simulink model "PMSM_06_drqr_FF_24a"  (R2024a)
settings: Solver=ode45  StartTime=0.0  StopTime=0.1  MaxStep=1e-4  RelTol=1e-4  AbsTol=1e-4  EnableMultiTasking=on
undefined symbols (not defined in the file): by, established, Flux, linkage, magnets, V
libraries: spsControlledVoltageSourceLib x3, spsCurrentMeasurementLib x3, slpidlib x2, spsPermanentMagnetSynchronousMachineLib x1, spspowerguiLib x1

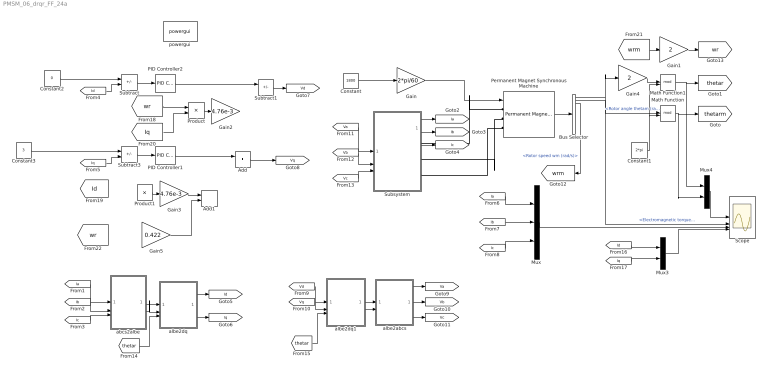
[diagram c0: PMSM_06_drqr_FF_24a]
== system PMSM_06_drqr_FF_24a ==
  Add : Sum
  Add1 : Sum
  Bus Selector : BusSelector  OutputSignals=Rotor angle thetam (rad),Electromagnetic torque Te (N*m),Rotor speed wm (rad/s)
  Constant : Constant  Value=1800
  Constant1 : Constant  Value=2*pi
  Constant2 : Constant  Value=0
  Constant3 : Constant  Value=3
  Gain : Gain  Gain=2*pi/60
  Gain1 : Gain  Gain=2
  Gain2 : Gain  Gain=4.76e-3
  Gain3 : Gain  Gain=4.76e-3
  Gain4 : Gain  Gain=2
  Gain5 : Gain  Gain=0.422
  Math Function : Math  Operator=mod  SignedPower=on
  Math Function1 : Math  Operator=mod  SignedPower=on
  Mux : Mux  Inputs=3
  Mux3 : Mux  Inputs=2
  Mux4 : Mux  Inputs=2
  PID Controller1 : slpidlib/PID Controller  Controller=PI  Form=Parallel  TimeDomain=Continuous-time  UseExternalTs=off  SampleTime=1  IntegratorMethod=Forward Euler  FilterMethod=Forward Euler  ControllerParametersSource=internal  P=14.95  I=1328.9  UseKiTs=off  D=0  UseExternalDerivativeSource=off  N=100  UseFilter=on  TunerSelectOption=Transfer Function Based (PID Tuner App)  InitialConditionSource=internal  InitialConditionForIntegrator=0  InitialConditionForFilter=0  DifferentiatorICPrevScaledInput=0  ExternalReset=none  TrackingMode=off  Kt=1  LimitOutput=off  SatLimitsSource=internal  UpperSaturationLimit=inf  LowerSaturationLimit=-inf  LinearizeAsGain=on  AntiWindupMode=none  Kb=1  LimitIntegrator=off  UpperIntegratorSaturationLimit=inf  LowerIntegratorSaturationLimit=-inf  POutMin=[]  POutMax=[]  IOutMin=[]  IOutMax=[]  DOutMin=[]  DOutMax=[]  NOutMin=[]  NOutMax=[]  SumOutMin=[]  SumOutMax=[]  SaturationOutMin=[]  SaturationOutMax=[]  PParamMin=[]  PParamMax=[]  IParamMin=[]  IParamMax=[]  DParamMin=[]  DParamMax=[]  NParamMin=[]  NParamMax=[]  KbParamMin=[]  KbParamMax=[]  KtParamMin=[]  KtParamMax=[]  KbOutMin=[]  KbOutMax=[]  KtOutMin=[]  KtOutMax=[]  IntegratorOutMin=[]  IntegratorOutMax=[]  FilterOutMin=[]  FilterOutMax=[]  SumI1OutMin=[]  SumI1OutMax=[]  SumI2OutMin=[]  SumI2OutMax=[]  SumI3OutMin=[]  SumI3OutMax=[]  SumI4OutMin=[]  SumI4OutMax=[]  SumDOutMin=[]  SumDOutMax=[]  DifferentiatorOutMin=[]  DifferentiatorOutMax=[]  FilterDiffOutCoefMin=[]  FilterDiffOutCoefMax=[]  ReciprocalOutMin=[]  ReciprocalOutMax=[]  SumDenOutMin=[]  SumDenOutMax=[]  SumNumOutMin=[]  SumNumOutMax=[]  DivideOutMin=[]  DivideOutMax=[]  UdiffTsProdOutMin=[]  UdiffTsProdOutMax=[]  NTsProdOutMin=[]  NTsProdOutMax=[]  UintegralTsProdOutMin=[]  UintegralTsProdOutMax=[]  UngainTsProdOutMin=[]  UngainTsProdOutMax=[]  ClampingZeroOutDataTypeStr=Inherit: Inherit via back propagation  ClampingZeroOutMin=[]  ClampingZeroOutMax=[]  FilterDenConstantOutDataTypeStr=Inherit: Inherit via back propagation  FilterDenConstantOutMin=[]  FilterDenConstantOutMax=[]  PCopyOutDataTypeStr=Inherit: Inherit via back propagation  PCopyOutMin=[]  PCopyOutMax=[]  NCopyOutDataTypeStr=Inherit: Inherit via back propagation  NCopyOutMin=[]  NCopyOutMax=[]  IntegratorContinuousStateAttributes=''  IntegratorStateMustResolveToSignalObject=off  IntegratorRTWStateStorageClass=Auto  FilterContinuousStateAttributes=''  FilterStateMustResolveToSignalObject=off  FilterRTWStateStorageClass=Auto  ParallelPVariant=InternalParameters  IdealPVariant=Disabled  IVariant=InternalParameters  DVariant=Disabled  IntegratorVariant=Continuous  SatVariant=Disabled  AWVariant=Passthrough  PCopyVariant=Disabled  TRVariant=Disabled  FdbkBlocksVariant=Forward  IdealPFdbkVariant=Disabled  SatFdbkVariant=Disabled  DerivativeFilterVariant=Disabled  NVariant=Disabled  NCopyVariant=Disabled_SignalSpec  FilterICVariant=Disabled  IntegratorICVariant=InternalICs  ExternalResetVariant=Disabled  TRSumVariant=Passthrough  SumFdbkVariant=Disabled  SumVariant=Sum_PI  TsampFilterVariant=InternalTs  TsampNgainVariant=Passthrough  TsampIntegralVariant=Disabled_SignalSpec  ExternalSaturationOutDataTypeStr=Inherit: Same as second input  DerivativeSourceVariant=Disabled
  PID Controller2 : slpidlib/PID Controller  Controller=PI  Form=Parallel  TimeDomain=Continuous-time  UseExternalTs=off  SampleTime=1  IntegratorMethod=Forward Euler  FilterMethod=Forward Euler  ControllerParametersSource=internal  P=14.95  I=1328.9  UseKiTs=off  D=0  UseExternalDerivativeSource=off  N=100  UseFilter=on  TunerSelectOption=Transfer Function Based (PID Tuner App)  InitialConditionSource=internal  InitialConditionForIntegrator=0  InitialConditionForFilter=0  DifferentiatorICPrevScaledInput=0  ExternalReset=none  TrackingMode=off  Kt=1  LimitOutput=off  SatLimitsSource=internal  UpperSaturationLimit=inf  LowerSaturationLimit=-inf  LinearizeAsGain=on  AntiWindupMode=none  Kb=1  LimitIntegrator=off  UpperIntegratorSaturationLimit=inf  LowerIntegratorSaturationLimit=-inf  POutMin=[]  POutMax=[]  IOutMin=[]  IOutMax=[]  DOutMin=[]  DOutMax=[]  NOutMin=[]  NOutMax=[]  SumOutMin=[]  SumOutMax=[]  SaturationOutMin=[]  SaturationOutMax=[]  PParamMin=[]  PParamMax=[]  IParamMin=[]  IParamMax=[]  DParamMin=[]  DParamMax=[]  NParamMin=[]  NParamMax=[]  KbParamMin=[]  KbParamMax=[]  KtParamMin=[]  KtParamMax=[]  KbOutMin=[]  KbOutMax=[]  KtOutMin=[]  KtOutMax=[]  IntegratorOutMin=[]  IntegratorOutMax=[]  FilterOutMin=[]  FilterOutMax=[]  SumI1OutMin=[]  SumI1OutMax=[]  SumI2OutMin=[]  SumI2OutMax=[]  SumI3OutMin=[]  SumI3OutMax=[]  SumI4OutMin=[]  SumI4OutMax=[]  SumDOutMin=[]  SumDOutMax=[]  DifferentiatorOutMin=[]  DifferentiatorOutMax=[]  FilterDiffOutCoefMin=[]  FilterDiffOutCoefMax=[]  ReciprocalOutMin=[]  ReciprocalOutMax=[]  SumDenOutMin=[]  SumDenOutMax=[]  SumNumOutMin=[]  SumNumOutMax=[]  DivideOutMin=[]  DivideOutMax=[]  UdiffTsProdOutMin=[]  UdiffTsProdOutMax=[]  NTsProdOutMin=[]  NTsProdOutMax=[]  UintegralTsProdOutMin=[]  UintegralTsProdOutMax=[]  UngainTsProdOutMin=[]  UngainTsProdOutMax=[]  ClampingZeroOutDataTypeStr=Inherit: Inherit via back propagation  ClampingZeroOutMin=[]  ClampingZeroOutMax=[]  FilterDenConstantOutDataTypeStr=Inherit: Inherit via back propagation  FilterDenConstantOutMin=[]  FilterDenConstantOutMax=[]  PCopyOutDataTypeStr=Inherit: Inherit via back propagation  PCopyOutMin=[]  PCopyOutMax=[]  NCopyOutDataTypeStr=Inherit: Inherit via back propagation  NCopyOutMin=[]  NCopyOutMax=[]  IntegratorContinuousStateAttributes=''  IntegratorStateMustResolveToSignalObject=off  IntegratorRTWStateStorageClass=Auto  FilterContinuousStateAttributes=''  FilterStateMustResolveToSignalObject=off  FilterRTWStateStorageClass=Auto  ParallelPVariant=InternalParameters  IdealPVariant=Disabled  IVariant=InternalParameters  DVariant=Disabled  IntegratorVariant=Continuous  SatVariant=Disabled  AWVariant=Passthrough  PCopyVariant=Disabled  TRVariant=Disabled  FdbkBlocksVariant=Forward  IdealPFdbkVariant=Disabled  SatFdbkVariant=Disabled  DerivativeFilterVariant=Disabled  NVariant=Disabled  NCopyVariant=Disabled_SignalSpec  FilterICVariant=Disabled  IntegratorICVariant=InternalICs  ExternalResetVariant=Disabled  TRSumVariant=Passthrough  SumFdbkVariant=Disabled  SumVariant=Sum_PI  TsampFilterVariant=InternalTs  TsampNgainVariant=Passthrough  TsampIntegralVariant=Disabled_SignalSpec  ExternalSaturationOutDataTypeStr=Inherit: Same as second input  DerivativeSourceVariant=Disabled
  Permanent Magnet Synchronous Machine : spsPermanentMagnetSynchronousMachineLib/Permanent Magnet Synchronous Machine  NbPhases=3  FluxDistribution=Sinusoidal  RotorType=Round  MechanicalLoad=Speed w  PresetModel=No  ShowDetailedParameters=on  MeasurementBus=off  Resistance=0.423  Inductance=8.5e-3  dqInductances=[8.5e-3,8.5e-3]  La=0.00476  MachineConstant=Flux linkage established by magnets (V.s)  Flux=0.422  VoltageCst=153.0847  TorqueCst=1.266  Flat=120  Mechanical=[0.03 0.04 4 0]  PolePairs=2  InitialConditions=[0,0, 0,0]  InitialConditions5ph=[0 0 0 0 0 0]  RefAngle=Aligned with phase A axis (original Park)  IterativeDiscreteModel=Trapezoidal non iterative  TsBlock=-1  TsPowergui=0
  Product : Product
  Product1 : Product
  Scope : Scope  NumInputPorts=4
  Subsystem : Subsystem
  Subtract : Sum  Inputs=+-
  Subtract1 : Sum  Inputs=+-
  Subtract3 : Sum  Inputs=+-
  abcs2albe : Subsystem
  albe2abcs : Subsystem
  albe2dq : Subsystem
  albe2dq1 : Subsystem
  powergui : spspowerguiLib/powergui  Priority=1  SimulationMode=Continuous  SampleTime=50e-6  frequency=60  Iterations=50  frequencyindice=0  Pbase=100e6  ErrMax=1e-4  UnitsV=kV  UnitsW=MW  buscounter=0  FunctionMessages=off  echomessages=off  EnableUseOfTLC=off  CurrentSourceSwitches=off  DisableSnubberDevices=on  DisableRonSwitches=on  DisableVfSwitches=on  DisplayEquations=off  AutomaticDiscreteSolvers=off  SolverType=Tustin  Interpol=off  ExternalGateDelay=off  methode=off  Ts=0  x0status=blocks  SPID=on  SwTol=0  HookPort=off  NonlinearTolerance=1e-4  nMaxIteration=100  ContinueOnMaxIteration=off  RestoreLinks=warning  ResistiveCurrentMeasurement=off  Frange=[0:2:500]  Ylog=off  Xlog=on  ShowGrid=off  save=off  variable=ZData  structure=0  ZoomFFT=off  StartTime=0.0  cycles=1  DisplayStyle=1  fundamental=60  FreqAxis=off  MaxFrequency=1000  frequencyindicesteady=1  RmsSteady=1  display=off
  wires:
  Gain/1 -> Permanent Magnet Synchronous Machine/1
  Constant/1 -> Gain/1
  Subtract/1 -> PID Controller2/1
  Permanent Magnet Synchronous Machine/1 -> Bus Selector/1
  Mux/1 -> Scope/3
  Bus Selector/2 -> Scope/2  "<Electromagnetic torque Te (N*m)>"
  Bus Selector/1 -> Gain4/1, Math Function/1  "<Rotor angle thetam (rad)>"
  Constant1/1 -> Math Function1/2, Math Function/2
  Math Function/1 -> Mux4/2, [thetarm]
  Gain4/1 -> Math Function1/1
  Math Function1/1 -> Mux4/1, [thetar]
  Subtract3/1 -> PID Controller1/1
  Subsystem/1(Out1) -> [Ia]
  Subsystem/2(Out2) -> [Ib]
  Subsystem/3(Out3) -> [Ic]
  [Id] -> Subtract/2
  [Iq] -> Subtract3/2
  [Ia] -> Mux/1
  [Ib] -> Mux/2
  [Ic] -> Mux/3
  Mux3/1 -> Scope/4
  [Id] -> Mux3/1
  [Iq] -> Mux3/2
  Mux4/1 -> Scope/1
  albe2dq1/1(alpha) -> albe2abcs/1(alpha)
  albe2dq1/2(beta) -> albe2abcs/2(beta)
  albe2abcs/1(as) -> [Va]
  albe2abcs/2(bs) -> [Vb]
  albe2abcs/3(cs) -> [Vc]
  [Ia] -> abcs2albe/1(as)
  [Ib] -> abcs2albe/2(bs)
  [Ic] -> abcs2albe/3(cs)
  [Vc] -> Subsystem/3(In3)
  [Vb] -> Subsystem/2(In2)
  [Va] -> Subsystem/1(In1)
  Bus Selector/3 -> [wrm]  "<Rotor speed wm (rad/s)>"
  abcs2albe/1(alpha) -> albe2dq/1(alpha)
  abcs2albe/2(beta) -> albe2dq/2(beta)
  albe2dq/1(d) -> [Id]
  albe2dq/2(q) -> [Iq]
  [thetar] -> albe2dq/3(thetar)
  [Vq] -> albe2dq1/2(q)
  [Vd] -> albe2dq1/1(d)
  [thetar] -> albe2dq1/3(thetar)
  Constant3/1 -> Subtract3/1
  Constant2/1 -> Subtract/1
  PID Controller1/1 -> Add/1
  Add/1 -> [Vq]
  PID Controller2/1 -> Subtract1/1
  Subtract1/1 -> [Vd]
  [wrm] -> Gain1/1
  Gain1/1 -> [wr]
  Product/1 -> Gain2/1
  [Iq] -> Product/2
  [wr] -> Product/1
  Product1/1 -> Gain3/1
  Gain3/1 -> Add1/1
  Gain5/1 -> Add1/2
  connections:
  Subsystem/RConn1 -- Permanent Magnet Synchronous Machine/LConn1
  Permanent Magnet Synchronous Machine/LConn2 -- Subsystem/RConn2
  Subsystem/RConn3 -- Permanent Magnet Synchronous Machine/LConn3

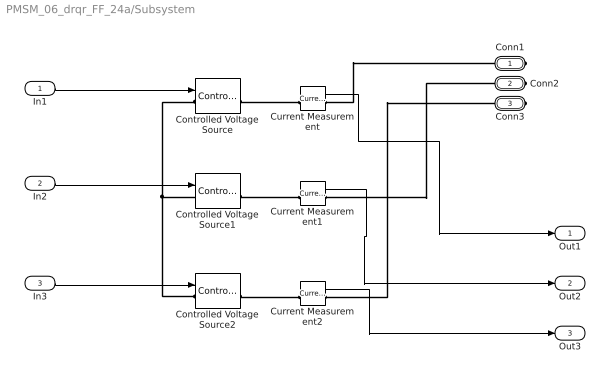
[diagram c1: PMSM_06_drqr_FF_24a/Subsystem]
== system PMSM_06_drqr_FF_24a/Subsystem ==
  In1 : Inport
  In2 : Inport  Port=2
  In3 : Inport  Port=3
  Controlled Voltage Source : spsControlledVoltageSourceLib/Controlled Voltage Source  Initialize=on  Source_Type=AC  Amplitude=0  Phase=0  Frequency=0  Measurements=None
  Controlled Voltage Source1 : spsControlledVoltageSourceLib/Controlled Voltage Source  Initialize=on  Source_Type=AC  Amplitude=0  Phase=0  Frequency=0  Measurements=None
  Controlled Voltage Source2 : spsControlledVoltageSourceLib/Controlled Voltage Source  Initialize=on  Source_Type=AC  Amplitude=0  Phase=0  Frequency=0  Measurements=None
  Current Measurement : spsCurrentMeasurementLib/Current Measurement  PhasorSimulation=off  OutputType=Complex  PSBequivalent=0
  Current Measurement1 : spsCurrentMeasurementLib/Current Measurement  PhasorSimulation=off  OutputType=Complex  PSBequivalent=0
  Current Measurement2 : spsCurrentMeasurementLib/Current Measurement  PhasorSimulation=off  OutputType=Complex  PSBequivalent=0
  Conn1 : PMIOPort  Side=Right
  Conn2 : PMIOPort  Port=2  Side=Right
  Conn3 : PMIOPort  Port=3  Side=Right
  Out1 : Outport
  Out2 : Outport  Port=2
  Out3 : Outport  Port=3
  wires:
  Current Measurement1/1 -> Out2/1
  In3/1 -> Controlled Voltage Source2/1
  In2/1 -> Controlled Voltage Source1/1
  In1/1 -> Controlled Voltage Source/1
  Current Measurement2/1 -> Out3/1
  Current Measurement/1 -> Out1/1
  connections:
  Current Measurement/RConn1 -- Conn1/RConn1
  Controlled Voltage Source/LConn1 -- Controlled Voltage Source1/LConn1 -- Controlled Voltage Source2/LConn1
  Controlled Voltage Source/RConn1 -- Current Measurement/LConn1
  Conn2/RConn1 -- Current Measurement1/RConn1
  Current Measurement2/RConn1 -- Conn3/RConn1
  Controlled Voltage Source1/RConn1 -- Current Measurement1/LConn1
  Controlled Voltage Source2/RConn1 -- Current Measurement2/LConn1

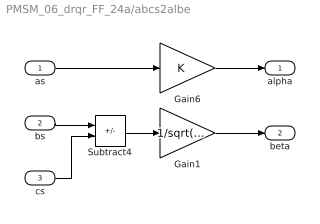
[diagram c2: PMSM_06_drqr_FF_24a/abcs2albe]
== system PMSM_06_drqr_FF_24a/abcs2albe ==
  as : Inport
  bs : Inport  Port=2
  cs : Inport  Port=3
  Gain1 : Gain  Gain=1/sqrt(3)
  Gain6 : Gain
  Subtract4 : Sum  Inputs=+-
  alpha : Outport
  beta : Outport  Port=2
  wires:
  bs/1 -> Subtract4/1
  as/1 -> Gain6/1
  cs/1 -> Subtract4/2
  Gain1/1 -> beta/1
  Subtract4/1 -> Gain1/1
  Gain6/1 -> alpha/1

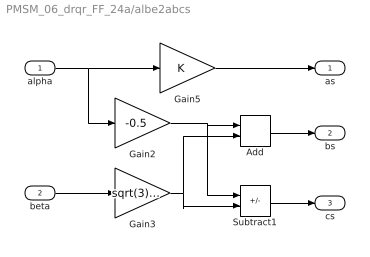
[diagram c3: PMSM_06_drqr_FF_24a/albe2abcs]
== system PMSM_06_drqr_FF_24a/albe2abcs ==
  alpha : Inport
  beta : Inport  Port=2
  Add : Sum
  Gain2 : Gain  Gain=-0.5
  Gain3 : Gain  Gain=sqrt(3)/2
  Gain5 : Gain
  Subtract1 : Sum  Inputs=+-
  as : Outport
  bs : Outport  Port=2
  cs : Outport  Port=3
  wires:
  alpha/1 -> Gain2/1, Gain5/1
  Gain3/1 -> Subtract1/2, Add/2
  Gain2/1 -> Subtract1/1, Add/1
  Add/1 -> bs/1
  Subtract1/1 -> cs/1
  beta/1 -> Gain3/1
  Gain5/1 -> as/1

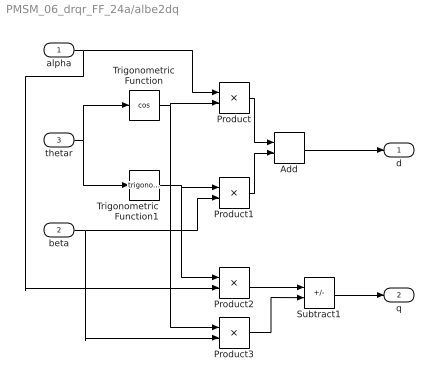
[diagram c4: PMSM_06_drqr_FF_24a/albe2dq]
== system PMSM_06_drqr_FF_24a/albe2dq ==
  alpha : Inport
  beta : Inport  Port=2
  thetar : Inport  Port=3
  Add : Sum
  Product{,1..3} (4 alike) : Product
  Subtract1 : Sum  Inputs=-+
  Trigonometric Function : Trigonometry  Operator=cos
  Trigonometric Function1 : Trigonometry
  d : Outport
  q : Outport  Port=2
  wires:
  thetar/1 -> Trigonometric Function/1, Trigonometric Function1/1
  Trigonometric Function/1 -> Product3/1, Product/2
  Trigonometric Function1/1 -> Product2/1, Product1/1
  beta/1 -> Product3/2, Product1/2
  Product/1 -> Add/1
  Product1/1 -> Add/2
  Add/1 -> d/1
  Subtract1/1 -> q/1
  alpha/1 -> Product/1, Product2/2
  Product2/1 -> Subtract1/1
  Product3/1 -> Subtract1/2

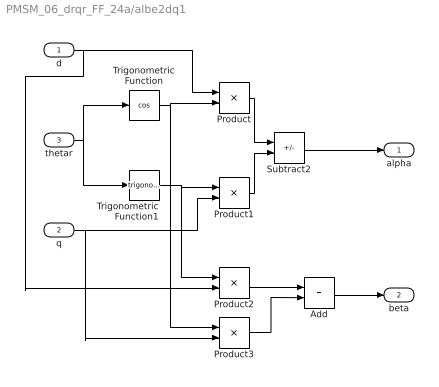
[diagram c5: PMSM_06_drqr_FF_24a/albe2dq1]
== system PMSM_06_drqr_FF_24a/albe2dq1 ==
  d : Inport
  q : Inport  Port=2
  thetar : Inport  Port=3
  Add : Sum
  Product{,1..3} (4 alike) : Product
  Subtract2 : Sum  Inputs=+-
  Trigonometric Function : Trigonometry  Operator=cos
  Trigonometric Function1 : Trigonometry
  alpha : Outport
  beta : Outport  Port=2
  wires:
  Product3/1 -> Add/2
  Product2/1 -> Add/1
  d/1 -> Product2/2, Product/1
  Add/1 -> beta/1
  Subtract2/1 -> alpha/1
  Product1/1 -> Subtract2/2
  Product/1 -> Subtract2/1
  q/1 -> Product1/2, Product3/2
  Trigonometric Function1/1 -> Product1/1, Product2/1
  Trigonometric Function/1 -> Product/2, Product3/1
  thetar/1 -> Trigonometric Function1/1, Trigonometric Function/1
